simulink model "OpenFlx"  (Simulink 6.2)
settings: Solver=ode45  StartTime=0.0  StopTime=10.0  RelTol=1e-3
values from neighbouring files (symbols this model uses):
  Av2 = Avn    [run3.m]
  Bv2 = Bvn    [run3.m]
  Cv2 = Cvn    [run3.m]
  Dv2 = Dvn    [run3.m]
  Kp = om^2*Iy/(l*T)    (= 0.554556771732)    [run.m]    (also in run3.m = 0.554540604935)
  Kr = 2*0.85*om*Iy/(l*T)    (= 1.03530256089)    [run.m]    (also in run3.m = 1.03527237908)
  wd = 7    [run.m]    (also in run3.m)
  wd2 = 16    [run.m]    (also in run3.m)
  wf = 9    [run.m]    (also in run3.m)
  wn = 7.4    [run.m]    (also in run3.m)
  wn2 = 16.8    [run.m]    (also in run3.m)
  zd = 0.2    [run.m]    (also in run3.m)
  zd2 = 0.2    [run.m]    (also in run3.m)
  zn = 0.02    [run.m]    (also in run3.m)
  zn2 = 0.015    [run.m]    (also in run3.m)
undefined symbols (not defined in the file or in its folder): Aa, Ba, Ca, Da

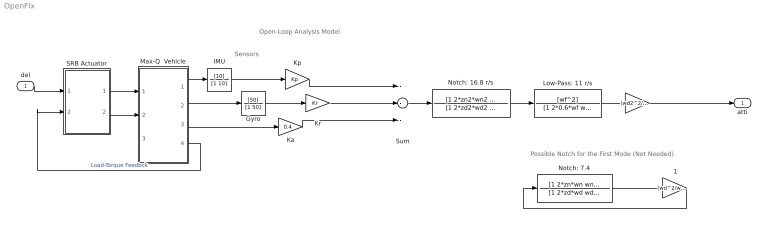
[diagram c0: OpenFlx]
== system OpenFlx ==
  note: Sensors
  note: Open-Loop Analysis Model
  note: Possible Notch for the First Mode (Not Needed)
  del : Inport  Port=1  LatchInput=off
  " " : Gain  Gain=(wd2^2/wn2^2)
  " 1" : Gain  Gain=(wd^2/wn^2)*(wd2^2/wn2^2)
  Gyro : TransferFcn  Numerator=[50]  Denominator=[1 50]
  IMU : TransferFcn  Numerator=[10]  Denominator=[1 10]
  Ka : Gain  Gain=0.4
  Kp : Gain  Gain=Kp
  Kr : Gain  Gain=Kr
  Low-Pass: 11 r/s : TransferFcn  Numerator=[wf^2]  Denominator=[1 2*0.6*wf wf^2]
  Max-Q  Vehicle : Subsystem
  Notch: 16.8 r/s : TransferFcn  Numerator=[1 2*zn2*wn2 wn2^2]  Denominator=[1 2*zd2*wd2 wd2^2]
  Notch: 7.4 : TransferFcn  Numerator=[1 2*zn*wn wn^2]  Denominator=[1 2*zd*wd wd^2]
  SRB Actuator : Subsystem
  Sum : Sum  Inputs=---
  atti : Outport
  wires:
  SRB Actuator/1(delto) -> Max-Q  Vehicle/1(delta)
  Kp/1 -> Sum/1
  Kr/1 -> Sum/2
  Max-Q  Vehicle/1(Theta) -> IMU/1
  IMU/1 -> Kp/1
  Max-Q  Vehicle/2(q-flx) -> Gyro/1
  Sum/1 -> Notch: 16.8 r/s/1
  Low-Pass: 11 r/s/1 -> " "/1
  Gyro/1 -> Kr/1
  del/1 -> SRB Actuator/1(delti)
  Max-Q  Vehicle/3(alflex) -> Ka/1
  Ka/1 -> Sum/3
  Notch: 16.8 r/s/1 -> Low-Pass: 11 r/s/1
  " "/1 -> atti/1
  SRB Actuator/2(delt-dd) -> Max-Q  Vehicle/2(delt-dd)
  Max-Q  Vehicle/4(TL) -> SRB Actuator/2(Ld-Tq)  "Load-Torque Feedbck"
  Notch: 7.4/1 -> " 1"/1
  " 1"/1 -> Notch: 7.4/1

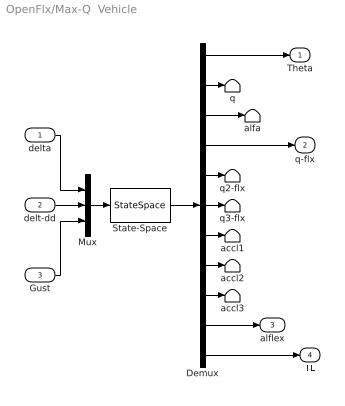
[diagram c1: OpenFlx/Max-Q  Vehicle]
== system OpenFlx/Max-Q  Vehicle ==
  delta : Inport  Port=1  LatchInput=off
  delt-dd : Inport  Port=2  LatchInput=off
  Gust : Inport  Port=3  LatchInput=off
  Demux : Demux  Outputs=11
  Mux : Mux  Inputs=3
  State-Space : StateSpace  A=Av2  B=Bv2  C=Cv2  D=Dv2
  accl1 : Terminator
  accl2 : Terminator
  accl3 : Terminator
  alfa : Terminator
  q : Terminator
  q2-flx : Terminator
  q3-flx : Terminator
  Theta : Outport
  q-flx : Outport  Port=2
  alflex : Outport  Port=3
  TL : Outport  Port=4
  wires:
  Mux/1 -> State-Space/1
  delta/1 -> Mux/1
  delt-dd/1 -> Mux/2
  Gust/1 -> Mux/3
  Demux/1 -> Theta/1
  Demux/4 -> q-flx/1
  Demux/8 -> accl2/1
  Demux/2 -> q/1
  Demux/5 -> q2-flx/1
  Demux/11 -> TL/1
  State-Space/1 -> Demux/1
  Demux/6 -> q3-flx/1
  Demux/9 -> accl3/1
  Demux/3 -> alfa/1
  Demux/10 -> alflex/1
  Demux/7 -> accl1/1

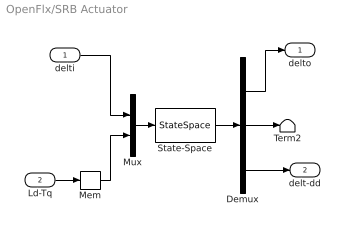
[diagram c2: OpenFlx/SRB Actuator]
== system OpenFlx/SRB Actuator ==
  delti : Inport  Port=1  LatchInput=off
  Ld-Tq : Inport  Port=2  LatchInput=off
  Demux : Demux  Outputs=3
  Mem : Memory
  Mux : Mux  Inputs=2
  State-Space : StateSpace  A=Aa  B=Ba  C=Ca  D=Da
  Term2 : Terminator
  delto : Outport
  delt-dd : Outport  Port=2
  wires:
  Mux/1 -> State-Space/1
  State-Space/1 -> Demux/1
  Demux/1 -> delto/1
  delti/1 -> Mux/1
  Ld-Tq/1 -> Mem/1
  Demux/3 -> delt-dd/1
  Demux/2 -> Term2/1
  Mem/1 -> Mux/2
